| TEXAS INSTRUMENTS INCORPORATED
| Standard Linear and Logic Group
| IBIS Model of SN74CBT16212A
| 24-BIT FET BUS-EXCHANGE SWITCHES
| This file contains package information for the following:
|  TVSOP 56-pin (DGV) package as [Component] CBT16212A_DGV
|  SSOP 56-pin (DL) package as [Component] CBT16212A_DL
|  TSSOP 56-pin (DGG) package as [Component] CBT16212A_DGG
|  VFBGA 56-pin (GQL) package as [Component] CBT16212A_GQL
| This device can be powered at the following Vccs:
|  5 volt Vcc
|  4 volt Vcc
| This file provides unique models under the [Model Selector] for each Vcc.
| For operation at a specific Vcc, select the appropriate model after each
| [Model Selector] keyword.
[IBIS Ver]   3.2
[Comment char]  |_char
[File Name]   sn74cbt16212a.ibs
[File Rev]   1.1 | d_die
[Date]   August 26, 2002
[Source]   Data created from TI-SPICE simulations at TI-SLL.
[Notes]   The following is an IBIS list for the CBT16212A_DL.
   Please contact sllibis@ti.com with questions and
   comments concerning SLL IBIS models.
   -Power-clamp data has been deleted since there is no
   power-clamp diode in the device.
   -Non-monotonic data due to device characteristics.
[Disclaimer] Property of Texas Instruments Incorporated.  Unauthorized
   reproduction and/or distribution is strictly prohibited.
   This product is protected under copyright law.
   Created  2002, (C) Copyright  2002, Texas Instruments
   Incorporated, All Rights Reserved
   UNLESS THERE IS A SIGNED, WRITTEN AGREEMENT TO THE
   CONTRARY, TEXAS INSTRUMENTS (TI) IS PROVIDING THE IBIS
   MODELS  AND WITHOUT ANY WARRANTY, EXPRESSED OR
   IMPLIED.  TI assumes no liability for:
   1) the accuracy of the IBIS models provided to your
   company;
   2) the proper functioning of these IBIS Models in your
   design or for any resulting applications; or
   3) infringement of patents, copyrights or intellectual
   property rights resulting from your use of these IBIS
   models.
   TI provides IBIS Models as a service to our customers.
   You and your company shall not distribute, sell or give
   these models to anyone else without prior written
   permission from TI.
   TI reserves the right to make changes to our products or
   to discontinue any semiconductor product or service
   without notice, and advises our customers to obtain the
   latest version of relevant information to verify, before
   placing orders, that the information being relied on is
   current.
   Please be aware that your receipt and use of the IBIS
   information provided shall serve as acceptance of these
   terms and conditions.  If you do not accept these terms,
   you should return or destroy the IBIS models and any
   other accompanying information immediately.
| Component CBT16212A_DGV 56-pin TVSOP
[Component]   CBT16212A_DGV
[Manufacturer]   Texas Instruments, Inc.
[Package]
|   typ   min   max
R_pkg   6.300e-02   5.000e-02   8.600e-02
L_pkg   2.945e-09   2.392e-09   3.938e-09
C_pkg   3.910e-13   2.710e-13   5.880e-13
[Pin]   signal_name   model_name   R_pin   L_pin   C_pin
1   S0   CBT16212A_IN   6.800e-02   3.933e-09   5.880e-13
2   1A1   CBT16212A_IO   6.800e-02   3.569e-09   5.860e-13
3   1A2   CBT16212A_IO   7.600e-02   3.464e-09   5.150e-13
4   2A1   CBT16212A_IO   8.600e-02   3.451e-09   4.580e-13
5   2A2   CBT16212A_IO   8.200e-02   3.278e-09   4.260e-13
6   3A1   CBT16212A_IO   7.700e-02   3.143e-09   3.870e-13
7   3A2   CBT16212A_IO   6.900e-02   2.971e-09   4.010e-13
8   GND   GND   5.000e-02   2.787e-09   3.790e-13
9   4A1   CBT16212A_IO   5.100e-02   2.686e-09   3.200e-13
10   4A2   CBT16212A_IO   5.200e-02   2.607e-09   3.160e-13
11   5A1   CBT16212A_IO   5.300e-02   2.497e-09   2.970e-13
12   5A2   CBT16212A_IO   5.400e-02   2.438e-09   2.920e-13
13   6A1   CBT16212A_IO   5.500e-02   2.412e-09   2.860e-13
14   6A2   CBT16212A_IO   5.500e-02   2.400e-09   2.730e-13
15   7A1   CBT16212A_IO   5.500e-02   2.402e-09   2.730e-13
16   7A2   CBT16212A_IO   5.400e-02   2.398e-09   2.840e-13
17   VCC   POWER   5.400e-02   2.407e-09   2.890e-13
18   8A1   CBT16212A_IO   5.300e-02   2.448e-09   2.930e-13
19   GND   GND   5.200e-02   2.548e-09   3.110e-13
20   8A2   CBT16212A_IO   5.100e-02   2.623e-09   3.160e-13
21   9A1   CBT16212A_IO   5.000e-02   2.725e-09   3.700e-13
22   9A2   CBT16212A_IO   6.500e-02   2.903e-09   3.940e-13
23   10A1   CBT16212A_IO   7.300e-02   3.086e-09   3.870e-13
24   10A2   CBT16212A_IO   8.200e-02   3.272e-09   4.280e-13
25   11A1   CBT16212A_IO   8.200e-02   3.394e-09   4.570e-13
26   11A2   CBT16212A_IO   7.100e-02   3.374e-09   5.080e-13
27   12A1   CBT16212A_IO   6.900e-02   3.572e-09   5.810e-13
28   12A2   CBT16212A_IO   6.900e-02   3.937e-09   5.740e-13
29   12B2   CBT16212A_IO   6.900e-02   3.923e-09   5.690e-13
30   12B1   CBT16212A_IO   6.800e-02   3.546e-09   5.740e-13
31   11B2   CBT16212A_IO   7.400e-02   3.422e-09   5.180e-13
32   11B1   CBT16212A_IO   8.100e-02   3.395e-09   4.680e-13
33   10B2   CBT16212A_IO   8.000e-02   3.255e-09   4.310e-13
34   10B1   CBT16212A_IO   7.100e-02   3.063e-09   3.860e-13
35   9B2   CBT16212A_IO   6.100e-02   2.878e-09   3.900e-13
36   9B1   CBT16212A_IO   5.000e-02   2.709e-09   3.640e-13
37   8B2   CBT16212A_IO   5.100e-02   2.607e-09   3.110e-13
38   GND   GND   5.100e-02   2.532e-09   3.060e-13
39   8B1   CBT16212A_IO   5.300e-02   2.440e-09   2.890e-13
40   7B2   CBT16212A_IO   5.300e-02   2.399e-09   2.860e-13
41   7B1   CBT16212A_IO   5.400e-02   2.392e-09   2.820e-13
42   6B2   CBT16212A_IO   5.500e-02   2.399e-09   2.710e-13
43   6B1   CBT16212A_IO   5.500e-02   2.395e-09   2.710e-13
44   5B2   CBT16212A_IO   5.500e-02   2.403e-09   2.830e-13
45   5B1   CBT16212A_IO   5.400e-02   2.421e-09   2.880e-13
46   4B2   CBT16212A_IO   5.300e-02   2.472e-09   2.920e-13
47   4B1   CBT16212A_IO   5.100e-02   2.569e-09   3.090e-13
48   3B2   CBT16212A_IO   5.100e-02   2.636e-09   3.130e-13
49   GND   GND   5.000e-02   2.739e-09   3.660e-13
50   3B1   CBT16212A_IO   6.500e-02   2.922e-09   3.900e-13
51   2B2   CBT16212A_IO   7.200e-02   3.076e-09   3.840e-13
52   2B1   CBT16212A_IO   8.100e-02   3.249e-09   4.300e-13
53   1B2   CBT16212A_IO   8.300e-02   3.400e-09   4.550e-13
54   1B1   CBT16212A_IO   7.300e-02   3.421e-09   5.060e-13
55   S2   CBT16212A_IN   6.900e-02   3.579e-09   5.780e-13
56   S1   CBT16212A_IN   6.900e-02   3.938e-09   5.810e-13
| Component CBT16212A_DL 56-pin SSOP
[Component]   CBT16212A_DL
[Manufacturer]   Texas Instruments, Inc.
[Package]
|   typ   min   max
R_pkg   5.500e-02   4.800e-02   6.700e-02
L_pkg   6.539e-09   4.802e-09   9.746e-09
C_pkg   1.880e-13   7.600e-14   5.170e-13
[Pin]   signal_name   model_name   R_pin   L_pin   C_pin
1   S0   CBT16212A_IN   6.400e-02   9.646e-09   5.130e-13
2   1A1   CBT16212A_IO   5.900e-02   8.723e-09   2.700e-13
3   1A2   CBT16212A_IO   5.900e-02   8.139e-09   2.230e-13
4   2A1   CBT16212A_IO   5.600e-02   7.554e-09   2.010e-13
5   2A2   CBT16212A_IO   5.400e-02   6.991e-09   1.950e-13
6   3A1   CBT16212A_IO   5.300e-02   6.659e-09   2.020e-13
7   3A2   CBT16212A_IO   5.500e-02   6.321e-09   2.070e-13
8   GND   GND   5.500e-02   5.942e-09   1.330e-13
9   4A1   CBT16212A_IO   5.700e-02   5.767e-09   1.320e-13
10   4A2   CBT16212A_IO   5.400e-02   5.459e-09   1.210e-13
11   5A1   CBT16212A_IO   5.100e-02   5.224e-09   1.400e-13
12   5A2   CBT16212A_IO   4.800e-02   5.088e-09   1.260e-13
13   6A1   CBT16212A_IO   5.000e-02   5.021e-09   9.600e-14
14   6A2   CBT16212A_IO   5.100e-02   4.802e-09   7.600e-14
15   7A1   CBT16212A_IO   5.100e-02   4.803e-09   7.600e-14
16   7A2   CBT16212A_IO   5.000e-02   5.021e-09   9.600e-14
17   VCC   POWER   4.800e-02   5.088e-09   1.260e-13
18   8A1   CBT16212A_IO   5.100e-02   5.224e-09   1.400e-13
19   GND   GND   5.400e-02   5.459e-09   1.210e-13
20   8A2   CBT16212A_IO   5.700e-02   5.768e-09   1.330e-13
21   9A1   CBT16212A_IO   5.500e-02   5.942e-09   1.330e-13
22   9A2   CBT16212A_IO   5.500e-02   6.320e-09   2.060e-13
23   10A1   CBT16212A_IO   5.300e-02   6.659e-09   2.030e-13
24   10A2   CBT16212A_IO   5.400e-02   6.991e-09   1.960e-13
25   11A1   CBT16212A_IO   5.600e-02   7.554e-09   2.010e-13
26   11A2   CBT16212A_IO   5.900e-02   8.139e-09   2.230e-13
27   12A1   CBT16212A_IO   5.900e-02   8.727e-09   2.700e-13
28   12A2   CBT16212A_IO   6.700e-02   9.746e-09   5.170e-13
29   12B2   CBT16212A_IO   6.300e-02   9.630e-09   5.110e-13
30   12B1   CBT16212A_IO   6.000e-02   8.751e-09   2.710e-13
31   11B2   CBT16212A_IO   6.000e-02   8.184e-09   2.250e-13
32   11B1   CBT16212A_IO   5.600e-02   7.543e-09   2.000e-13
33   10B2   CBT16212A_IO   5.400e-02   7.005e-09   1.960e-13
34   10B1   CBT16212A_IO   5.600e-02   6.714e-09   2.040e-13
35   9B2   CBT16212A_IO   5.800e-02   6.384e-09   2.080e-13
36   9B1   CBT16212A_IO   5.700e-02   5.976e-09   1.340e-13
37   8B2   CBT16212A_IO   5.700e-02   5.743e-09   1.300e-13
38   GND   GND   5.400e-02   5.468e-09   1.190e-13
39   8B1   CBT16212A_IO   5.500e-02   5.328e-09   1.420e-13
40   7B2   CBT16212A_IO   5.200e-02   5.189e-09   1.290e-13
41   7B1   CBT16212A_IO   5.200e-02   5.053e-09   9.600e-14
42   6B2   CBT16212A_IO   5.100e-02   4.825e-09   7.600e-14
43   6B1   CBT16212A_IO   5.400e-02   4.896e-09   7.800e-14
44   5B2   CBT16212A_IO   5.200e-02   5.093e-09   9.700e-14
45   5B1   CBT16212A_IO   5.100e-02   5.179e-09   1.280e-13
46   4B2   CBT16212A_IO   5.400e-02   5.314e-09   1.420e-13
47   4B1   CBT16212A_IO   5.500e-02   5.511e-09   1.210e-13
48   3B2   CBT16212A_IO   5.700e-02   5.771e-09   1.310e-13
49   GND   GND   5.600e-02   5.957e-09   1.330e-13
50   3B1   CBT16212A_IO   5.500e-02   6.320e-09   2.060e-13
51   2B2   CBT16212A_IO   5.200e-02   6.621e-09   2.000e-13
52   2B1   CBT16212A_IO   5.300e-02   6.973e-09   1.950e-13
53   1B2   CBT16212A_IO   5.700e-02   7.571e-09   2.020e-13
54   1B1   CBT16212A_IO   5.700e-02   8.097e-09   2.220e-13
55   S2   CBT16212A_IN   5.900e-02   8.723e-09   2.710e-13
56   S1   CBT16212A_IN   6.100e-02   9.560e-09   5.090e-13
| Component CBT16212A_DGG 56-pin TSSOP
[Component]   CBT16212A_DGG
[Manufacturer]   Texas Instruments, Inc.
[Package]
|   typ   min   max
R_pkg   4.500e-02   3.500e-02   6.200e-02
L_pkg   3.324e-09   2.403e-09   5.094e-09
C_pkg   5.640e-13   3.410e-13   9.140e-13
[Pin]   signal_name   model_name   R_pin   L_pin   C_pin
1   S0   CBT16212A_IN   6.200e-02   5.094e-09   8.560e-13
2   1A1   CBT16212A_IO   6.100e-02   4.621e-09   9.020e-13
3   1A2   CBT16212A_IO   6.000e-02   4.316e-09   8.020e-13
4   2A1   CBT16212A_IO   5.900e-02   3.968e-09   6.980e-13
5   2A2   CBT16212A_IO   5.700e-02   3.716e-09   6.490e-13
6   3A1   CBT16212A_IO   4.200e-02   3.517e-09   6.520e-13
7   3A2   CBT16212A_IO   4.100e-02   3.160e-09   5.700e-13
8   GND   GND   3.900e-02   2.981e-09   4.820e-13
9   4A1   CBT16212A_IO   3.900e-02   2.809e-09   4.470e-13
10   4A2   CBT16212A_IO   3.800e-02   2.715e-09   4.090e-13
11   5A1   CBT16212A_IO   4.100e-02   2.675e-09   3.910e-13
12   5A2   CBT16212A_IO   3.900e-02   2.536e-09   3.660e-13
13   6A1   CBT16212A_IO   3.900e-02   2.457e-09   3.480e-13
14   6A2   CBT16212A_IO   3.800e-02   2.411e-09   3.530e-13
15   7A1   CBT16212A_IO   3.900e-02   2.456e-09   3.550e-13
16   7A2   CBT16212A_IO   3.900e-02   2.471e-09   3.490e-13
17   VCC   POWER   4.000e-02   2.580e-09   3.700e-13
18   8A1   CBT16212A_IO   3.800e-02   2.651e-09   3.890e-13
19   GND   GND   3.800e-02   2.739e-09   4.110e-13
20   8A2   CBT16212A_IO   3.900e-02   2.838e-09   4.490e-13
21   9A1   CBT16212A_IO   3.800e-02   2.988e-09   4.840e-13
22   9A2   CBT16212A_IO   3.800e-02   3.105e-09   5.640e-13
23   10A1   CBT16212A_IO   4.000e-02   3.427e-09   6.380e-13
24   10A2   CBT16212A_IO   5.600e-02   3.654e-09   6.410e-13
25   11A1   CBT16212A_IO   5.700e-02   3.932e-09   7.000e-13
26   11A2   CBT16212A_IO   5.800e-02   4.257e-09   8.060e-13
27   12A1   CBT16212A_IO   5.700e-02   4.580e-09   9.140e-13
28   12A2   CBT16212A_IO   5.900e-02   5.038e-09   8.610e-13
29   12B2   CBT16212A_IO   6.000e-02   5.058e-09   8.580e-13
30   12B1   CBT16212A_IO   5.600e-02   4.543e-09   9.040e-13
31   11B2   CBT16212A_IO   5.700e-02   4.240e-09   8.030e-13
32   11B1   CBT16212A_IO   5.700e-02   3.929e-09   7.000e-13
33   10B2   CBT16212A_IO   5.600e-02   3.616e-09   6.370e-13
34   10B1   CBT16212A_IO   3.700e-02   3.368e-09   6.400e-13
35   9B2   CBT16212A_IO   3.600e-02   3.024e-09   5.630e-13
36   9B1   CBT16212A_IO   3.500e-02   2.876e-09   4.740e-13
37   8B2   CBT16212A_IO   3.500e-02   2.745e-09   4.440e-13
38   GND   GND   3.700e-02   2.683e-09   4.050e-13
39   8B1   CBT16212A_IO   3.800e-02   2.603e-09   3.820e-13
40   7B2   CBT16212A_IO   3.800e-02   2.510e-09   3.620e-13
41   7B1   CBT16212A_IO   3.600e-02   2.412e-09   3.410e-13
42   6B2   CBT16212A_IO   3.800e-02   2.416e-09   3.490e-13
43   6B1   CBT16212A_IO   3.700e-02   2.403e-09   3.490e-13
44   5B2   CBT16212A_IO   3.700e-02   2.429e-09   3.410e-13
45   5B1   CBT16212A_IO   3.600e-02   2.482e-09   3.580e-13
46   4B2   CBT16212A_IO   3.700e-02   2.615e-09   3.810e-13
47   4B1   CBT16212A_IO   3.500e-02   2.669e-09   4.020e-13
48   3B2   CBT16212A_IO   3.600e-02   2.763e-09   4.420e-13
49   GND   GND   3.600e-02   2.942e-09   4.780e-13
50   3B1   CBT16212A_IO   3.500e-02   3.053e-09   5.640e-13
51   2B2   CBT16212A_IO   3.600e-02   3.409e-09   6.410e-13
52   2B1   CBT16212A_IO   5.800e-02   3.698e-09   6.410e-13
53   1B2   CBT16212A_IO   5.900e-02   3.975e-09   6.970e-13
54   1B1   CBT16212A_IO   6.100e-02   4.327e-09   8.020e-13
55   S2   CBT16212A_IN   6.100e-02   4.624e-09   9.050e-13
56   S1   CBT16212A_IN   6.000e-02   5.063e-09   8.580e-13
| Component CBT16212A_GQL 56-pin VFBGA
[Component]   CBT16212A_GQL
[Manufacturer]   Texas Instruments, Inc.
[Package]
|   typ   min   max
R_pkg   6.500e-02   3.500e-02   9.700e-02
L_pkg   1.952e-09   1.000e-09   3.191e-09
C_pkg   2.830e-13   1.620e-13   4.340e-13
[Pin]   signal_name   model_name   R_pin   L_pin   C_pin
1   S0   CBT16212A_IN   3.600e-02   1.004e-09   1.760e-13
2   1A1   CBT16212A_IO   4.000e-02   1.191e-09   1.860e-13
3   1A2   CBT16212A_IO   4.700e-02   1.411e-09   2.090e-13
4   2A1   CBT16212A_IO   9.700e-02   3.191e-09   4.340e-13
5   2A2   CBT16212A_IO   7.400e-02   2.213e-09   3.290e-13
6   3A1   CBT16212A_IO   6.000e-02   1.712e-09   2.430e-13
7   3A2   CBT16212A_IO   8.500e-02   2.691e-09   3.680e-13
8   GND   GND   7.400e-02   2.160e-09   3.150e-13
9   4A1   CBT16212A_IO   6.000e-02   1.666e-09   2.470e-13
10   4A2   CBT16212A_IO   7.400e-02   2.121e-09   3.130e-13
11   5A1   CBT16212A_IO   9.100e-02   2.924e-09   3.970e-13
12   5A2   CBT16212A_IO   6.000e-02   1.619e-09   2.450e-13
13   6A1   CBT16212A_IO   6.900e-02   2.031e-09   2.880e-13
14   6A2   CBT16212A_IO   6.000e-02   1.583e-09   2.200e-13
15   7A1   CBT16212A_IO   6.000e-02   1.578e-09   2.200e-13
16   7A2   CBT16212A_IO   6.900e-02   2.017e-09   2.860e-13
17   VCC   POWER   6.000e-02   1.594e-09   2.410e-13
18   8A1   CBT16212A_IO   9.200e-02   2.917e-09   3.970e-13
19   GND   GND   7.500e-02   2.114e-09   3.150e-13
20   8A2   CBT16212A_IO   6.000e-02   1.632e-09   2.470e-13
21   9A1   CBT16212A_IO   7.000e-02   2.074e-09   3.070e-13
22   9A2   CBT16212A_IO   8.600e-02   2.664e-09   3.650e-13
23   10A1   CBT16212A_IO   6.000e-02   1.689e-09   2.490e-13
24   10A2   CBT16212A_IO   6.600e-02   2.152e-09   3.320e-13
25   11A1   CBT16212A_IO   8.700e-02   3.118e-09   4.230e-13
26   11A2   CBT16212A_IO   3.800e-02   1.303e-09   2.000e-13
27   12A1   CBT16212A_IO   3.500e-02   1.176e-09   1.830e-13
28   12A2   CBT16212A_IO   3.500e-02   1.007e-09   1.620e-13
29   12B2   CBT16212A_IO   3.500e-02   1.000e-09   1.620e-13
30   12B1   CBT16212A_IO   3.500e-02   1.154e-09   1.800e-13
31   11B2   CBT16212A_IO   4.100e-02   1.352e-09   2.040e-13
32   11B1   CBT16212A_IO   8.800e-02   3.137e-09   4.300e-13
33   10B2   CBT16212A_IO   7.400e-02   2.218e-09   3.340e-13
34   10B1   CBT16212A_IO   6.000e-02   1.683e-09   2.500e-13
35   9B2   CBT16212A_IO   8.500e-02   2.658e-09   3.720e-13
36   9B1   CBT16212A_IO   7.500e-02   2.149e-09   3.210e-13
37   8B2   CBT16212A_IO   6.000e-02   1.627e-09   2.480e-13
38   GND   GND   7.500e-02   2.113e-09   3.140e-13
39   8B1   CBT16212A_IO   9.200e-02   2.922e-09   3.960e-13
40   7B2   CBT16212A_IO   6.000e-02   1.594e-09   2.420e-13
41   7B1   CBT16212A_IO   6.900e-02   2.016e-09   2.880e-13
42   6B2   CBT16212A_IO   6.000e-02   1.580e-09   2.210e-13
43   6B1   CBT16212A_IO   6.000e-02   1.582e-09   2.200e-13
44   5B2   CBT16212A_IO   6.900e-02   2.026e-09   2.890e-13
45   5B1   CBT16212A_IO   6.000e-02   1.610e-09   2.450e-13
46   4B2   CBT16212A_IO   9.200e-02   2.933e-09   3.960e-13
47   4B1   CBT16212A_IO   7.500e-02   2.126e-09   3.110e-13
48   3B2   CBT16212A_IO   6.000e-02   1.641e-09   2.450e-13
49   GND   GND   7.300e-02   2.168e-09   3.190e-13
50   3B1   CBT16212A_IO   8.600e-02   2.675e-09   3.620e-13
51   2B2   CBT16212A_IO   6.000e-02   1.688e-09   2.430e-13
52   2B1   CBT16212A_IO   7.500e-02   2.281e-09   3.330e-13
53   1B2   CBT16212A_IO   9.500e-02   3.168e-09   4.240e-13
54   1B1   CBT16212A_IO   4.500e-02   1.418e-09   2.090e-13
55   S2   CBT16212A_IN   3.900e-02   1.216e-09   1.900e-13
56   S1   CBT16212A_IN   3.700e-02   1.029e-09   1.790e-13
[Series Switch Groups]
| Function Group States
On  1 /   | 1A1-1A2->1B1-1B2 S2 LOW S1 LOW S0 LOW
On  2 /   | 1A1-1A2->2B1-2B2 S2 LOW S1 HIGH S0 LOW
[Series Pin Mapping]   pin_2   model_name   function_table_group
2   54   CBT16212A_IO_50_S   1
| 2   54   CBT16212A_IO_40_S   1
3   53   CBT16212A_IO_50_S   1
| 3   53   CBT16212A_IO_40_S   1
2   52   CBT16212A_IO_50_S   2
| 2   52   CBT16212A_IO_40_S   2
3   51   CBT16212A_IO_50_S   2
| 3   51   CBT16212A_IO_40_S   2
| Model CBT16212A_IN
[Model Selector]   CBT16212A_IN
CBT16212A_IN_50   5 volt Vcc
CBT16212A_IN_40   4 volt Vcc
| Model CBT16212A_IO
[Model Selector]   CBT16212A_IO
CBT16212A_IO_50   5 volt Vcc
CBT16212A_IO_40   4 volt Vcc
| Model CBT16212A_IO_S
[Model Selector]   CBT16212A_IO_S
CBT16212A_IO_50_S   5 volt Vcc
CBT16212A_IO_40_S   4 volt Vcc
[Model]   CBT16212A_IO_50_S
Model_type  Series_switch
| variable   typ   min   max
C_comp   0   0   0
[Temperature Range]   40   100   -40
| Ambient temperature   25   85   -40
[Voltage range]   5   4.5   5.5
[On]
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[Off]
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[Model]   CBT16212A_IO_40_S
Model_type  Series_switch
| variable   typ   min   max
C_comp   0   0   0
[Temperature Range]   40   100   -40
| Ambient temperature   25   85   -40
[Voltage range]   4   4   4
[On]
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[Off]
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| Models and submodels in the file (6): CBT16212A_IN_50 (Input), CBT16212A_IN_40 (Input), CBT16212A_IO_50_S (Series_switch), CBT16212A_IO_50 (Terminator), CBT16212A_IO_40_S (Series_switch), CBT16212A_IO_40 (Terminator)
